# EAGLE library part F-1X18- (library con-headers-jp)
FEMALE HEADER
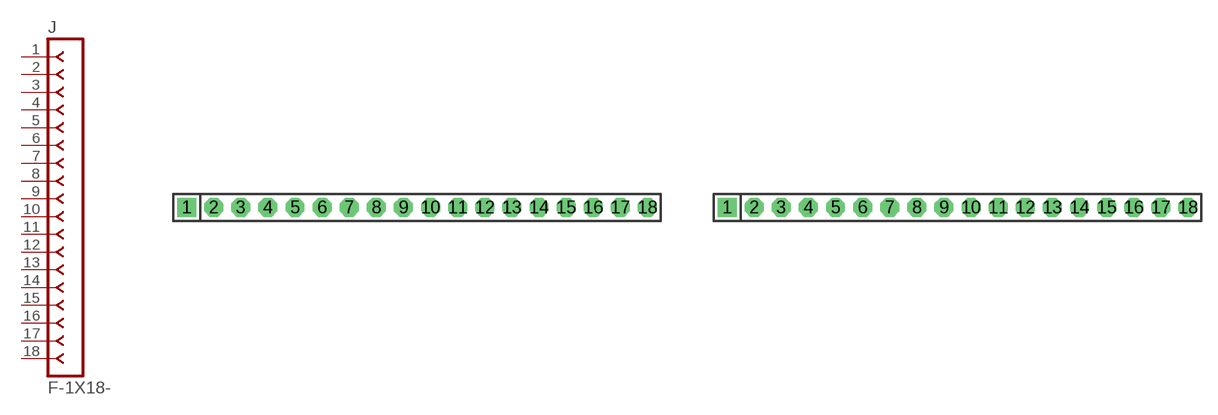
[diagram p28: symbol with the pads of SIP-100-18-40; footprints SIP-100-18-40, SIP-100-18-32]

Designator prefix J

## F-1X18-SIP-100-40  [SIP-100-18-40]
1  1  pas
2  2  pas
3  3  pas
4  4  pas
5  5  pas
6  6  pas
7  7  pas
8  8  pas
9  9  pas
10  10  pas
11  11  pas
12  12  pas
13  13  pas
14  14  pas
15  15  pas
16  16  pas
17  17  pas
18  18  pas

## F-1X18-SIP-100-32  [SIP-100-18-32]
Pads as for SIP-100-18-40

## F-1X18-SIP-100-32Y  [SIP-100-18-32Y]
Pads as for SIP-100-18-40

## F-1X18-SIP-100-40Y  [SIP-100-18-40Y]
Pads as for SIP-100-18-40

## F-1X18-KK-4455-B18  [KK-4455-B18]
Pads as for SIP-100-18-40

## F-1X18-KK-4455-C18  [KK-4455-C18]
Pads as for SIP-100-18-40

## F-1X18-KK-4455-A18  [KK-4455-A18]
Pads as for SIP-100-18-40

## Footprint SIP-100-18-40 (pad centres in mm)
SIP Header - 0.1", 40 mil drill
drill 1.016 pad 1.778 square: 1 -21.59,0
drill 1.016 pad 1.778 octagon: 2 -19.05,0; 3 -16.51,0; 4 -13.97,0; 5 -11.43,0; 6 -8.89,0; 7 -6.35,0; 8 -3.81,0; 9 -1.27,0; 10 1.27,0; 11 3.81,0; 12 6.35,0; 13 8.89,0; 14 11.43,0; 15 13.97,0; 16 16.51,0; 17 19.05,0; 18 21.59,0

## Footprint SIP-100-18-32 (pad centres in mm)
SIP Header - 0.1", 32 mil drill
drill 0.813 pad 1.778 square: 1 -21.59,0
drill 0.813 pad 1.778 octagon: 2 -19.05,0; 3 -16.51,0; 4 -13.97,0; 5 -11.43,0; 6 -8.89,0; 7 -6.35,0; 8 -3.81,0; 9 -1.27,0; 10 1.27,0; 11 3.81,0; 12 6.35,0; 13 8.89,0; 14 11.43,0; 15 13.97,0; 16 16.51,0; 17 19.05,0; 18 21.59,0

## Footprint SIP-100-18-32Y (pad centres in mm)
SIP Header - 0.1", 32 mil drill
drill 0.813 long: 1 -21.59,0; 2 -19.05,0; 3 -16.51,0; 4 -13.97,0; 5 -11.43,0; 6 -8.89,0; 7 -6.35,0; 8 -3.81,0; 9 -1.27,0; 10 1.27,0; 11 3.81,0; 12 6.35,0; 13 8.89,0; 14 11.43,0; 15 13.97,0; 16 16.51,0; 17 19.05,0; 18 21.59,0

## Footprint SIP-100-18-40Y (pad centres in mm)
SIP Header - 0.1", 40 mil drill
drill 1.016 long: 1 -21.59,0; 2 -19.05,0; 3 -16.51,0; 4 -13.97,0; 5 -11.43,0; 6 -8.89,0; 7 -6.35,0; 8 -3.81,0; 9 -1.27,0; 10 1.27,0; 11 3.81,0; 12 6.35,0; 13 8.89,0; 14 11.43,0; 15 13.97,0; 16 16.51,0; 17 19.05,0; 18 21.59,0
